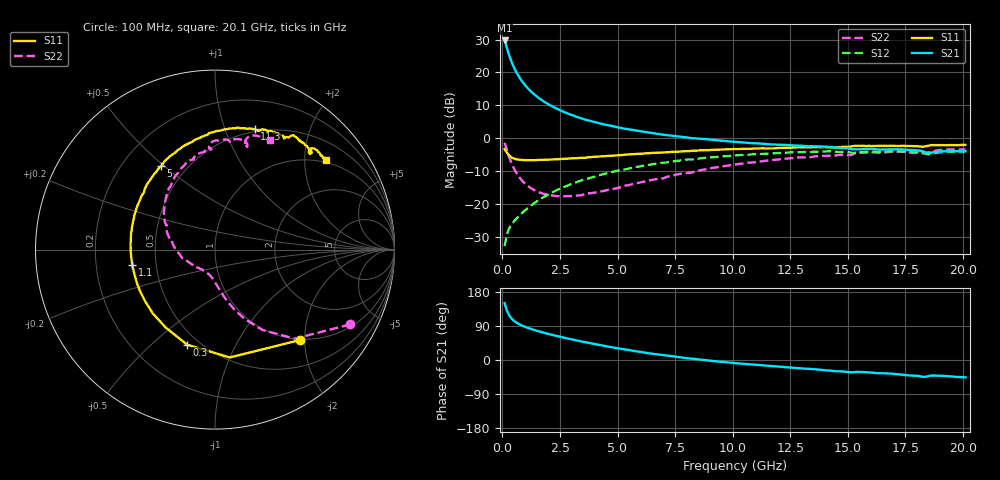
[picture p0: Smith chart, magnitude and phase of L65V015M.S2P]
!  Infineon Technologies AG
! BFR380L3 , PF131585-7, No.6, Th 09.10.01, soldered on pcb-board, measured with PP GSG850
!  Vce=5.0 V,  Ic=15.0 mA
! Common Emitter S-Parameters:  15. November 2001
#  GHz  S  MA  R  50
! f  S11  S21  S12  S22
! GHz  Mag  Ang  Mag  Ang  Mag  Ang  Mag  Ang
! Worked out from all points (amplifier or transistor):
!   201 points, 100 MHz to 20.1 GHz, reference 50 ohm
!   highest |S21| = 29.7 dB at 100 MHz (marker M1)
!   |S21| within 3 dB of that: start of sweep to 231.1 MHz
!   unconditionally stable (mu >= 1): 1.648 GHz to 4.421 GHz
!   at 3.4 GHz: K = 1.02, MAG = 8.6 dB, |S12| = -12.8 dB
!   at 10.1 GHz: K = 0.94, MSG = 2.1 dB, |S12| = -5.2 dB
!   at 20.1 GHz: K = 0.98, MSG = 0.1 dB, |S12| = -4.0 dB
!   S11 on the Smith chart (normalised r, x): 100 MHz: 0.98, -1.89; 300 MHz: 0.43, -0.66; 1.1 GHz: 0.36, -0.08; 5 GHz: 0.36, +0.49; 11.3 GHz: 0.47, +1.27; 20.1 GHz: 0.92, +2.53
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0.1  0.6902 -47.0  30.59 150.0  0.02325 68.5  0.8609 -29.0
0.2  0.6065 -82.2  23.46 129.9  0.03539 57.5  0.6663 -48.2
0.3  0.5522 -106.3  18.14 117.6  0.04355 53.6  0.5197 -59.5
0.4  0.5137 -122.4  14.53 109.4  0.04962 52.2  0.4204 -66.8
0.5  0.497 -134.1  12.03 103.6  0.05488 52.8  0.3529 -71.9
0.6  0.4845 -143.2  10.22 99.2  0.06003 53.8  0.3049 -75.8
0.7  0.4779 -150.5  8.889 95.5  0.0652 55.0  0.269 -78.9
0.8  0.4738 -156.3  7.841 92.3  0.07077 56.1  0.2421 -81.6
0.9  0.4701 -161.2  7.018 89.6  0.07622 57.1  0.2209 -83.9
1.1  0.4688 -169.4  5.81 84.9  0.08768 58.7  0.1915 -88.3
1.3  0.4683 -176.0  4.954 80.8  0.09936 59.8  0.1713 -92.2
1.5  0.4704 178.2  4.326 77.1  0.1112 60.5  0.1575 -96.0
2  0.4764 166.9  3.294 68.8  0.1419 60.6  0.1393 -105.7
2.6  0.4898 155.8  2.586 59.9  0.1788 59.2  0.1331 -117.8
3.5  0.5078 141.6  1.978 48.0  0.2347 55.4  0.1398 -134.3
5  0.5538 122.9  1.477 30.9  0.3244 46.9  0.1771 -162.9
6.8  0.6093 104.1  1.165 14.1  0.4207 35.2  0.2444 169.0
10.1  0.6913 79.1  0.8884 -8.3  0.5516 13.8  0.4021 132.5
11.3  0.707 71.7  0.8307 -14.5  0.5849 5.9  0.454 120.9
13.5  0.7344 61.2  0.76 -24.4  0.6261 -7.4  0.5283 102.6
16.8  0.7704 48.8  0.6828 -35.5  0.6352 -23.9  0.6238 80.1
20.1  0.7966 39.0  0.6425 -45.9  0.6284 -37.9  0.6833 63.2
